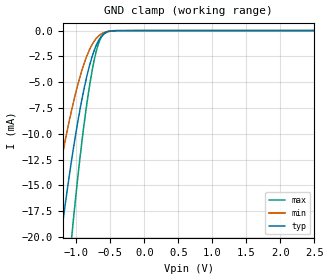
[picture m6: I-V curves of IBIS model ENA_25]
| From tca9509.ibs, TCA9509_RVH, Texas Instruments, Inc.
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[Model]   ENA_25
Model_type  Input
Vinl=0.15
Vinh=1.75
| variable   typ   min   max
C_comp   1.73pF   1.27pF   2.01pF
[Temperature Range]   40   100   -40
| Ambient temperature   25   85   -40
[Voltage range]   2.5   2.3   2.7
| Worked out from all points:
|   GND clamp passes 1 mA (typ) near -0.68 V on its own axis
[GND Clamp]
| ENA_25
|   Voltage   I(typ)   I(min)   I(max)
-2.5V     -109.9mA   -78.03mA   -160.4mA
-1.405V   -29.79mA   -19.62mA   -46.56mA
-1.21V    -19.12mA   -12.2mA    -30.31mA
-1.075V   -12.75mA   -7.861mA   -20.42mA
-1.055V   -11.89mA   -7.281mA   -19.07mA
-920mV    -6.722mA   -3.883mA   -10.84mA
-805mV    -3.354mA   -1.825mA   -5.303mA
-710mV    -1.465mA   -779.9uA   -2.066mA
-625mV    -513.9uA   -292.4uA   -560.9uA
-545mV    -136.8uA   -94.94uA   -106.9uA
-430mV    -13.52uA   -13.5uA    -5.631uA
2.5V      247.4pA    1.266nA    41.34pA
